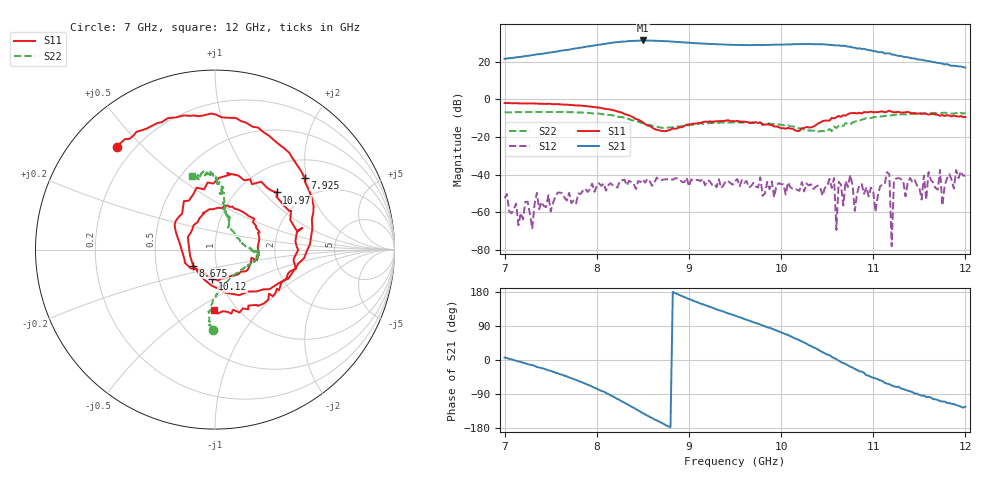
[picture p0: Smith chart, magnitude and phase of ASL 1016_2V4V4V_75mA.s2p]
!ASL 1016 Low Noise Amplifier S-parameter data 7-12 GHz
!Bias conditions Vd1=2V,Vd2=4V,Vd3=4V ; Ids = 75mA
!Agilent Technologies,N5230A,US43500341,A.06.01.05
!Agilent N5230A: A.06.01.05
!Date: Wednesday, October 04, 2006 13:12:58
!Correction: S11(Full 2 Port(1,2)) S21(Full 2 Port(1,2)) S12(Full 2 Port(1,2)) S22(Full 2 Port(1,2))
!S2P File: Measurements: S11, S21, S12, S22:
# Hz S  dB  R 50
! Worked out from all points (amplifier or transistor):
!   201 points, 7 GHz to 12 GHz, reference 50 ohm
!   highest |S21| = 31.2 dB at 8.5 GHz (marker M1)
!   |S21| within 3 dB of that: 7.931 GHz to 10.71 GHz (2.775 GHz wide, 29.8 % of centre)
!   unconditionally stable (mu >= 1): start of sweep to end of sweep
!   at 7.825 GHz: K = 3.33, MAG = 30.7 dB, |S12| = -50.2 dB
!   at 9.5 GHz: K = 2.53, MAG = 29.3 dB, |S12| = -43.5 dB
!   at 12 GHz: K = 5.47, MAG = 18.3 dB, |S12| = -40.5 dB
!   S11 on the Smith chart (normalised r, x): 7 GHz: 0.14, +0.42; 7.925 GHz: 1.43, +1.95; 8.675 GHz: 0.77, -0.14; 10.12 GHz: 0.92, -0.31; 10.97 GHz: 1.47, +1.20; 12 GHz: 0.79, -0.60
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7e9  -2.06 133.5  21.47 6.2  -52.53 164.1  -6.95 -91.5
7.425e9  -2.52 97.0  24.22 -22.6  -56.60 -127.1  -6.71 -91.3
7.85e9  -3.51 49.7  27.58 -59.5  -48.46 -156.3  -7.05 -92.2
7.925e9  -3.87 38.8  28.11 -67.4  -47.80 -179.0  -7.32 -93.1
8.075e9  -4.95 17.4  29.30 -83.5  -44.60 -153.8  -7.99 -94.6
8.2e9  -6.05 -5.5  30.20 -99.8  -46.45 156.1  -8.70 -94.6
8.35e9  -8.51 -36.0  30.85 -119.2  -43.22 160.0  -10.44 -92.8
8.5e9  -12.21 -77.2  31.17 -140.1  -42.46 155.5  -12.75 -83.8
8.675e9  -16.45 -143.5  30.99 -162.5  -42.69 140.4  -14.83 -63.3
8.825e9  -15.55 155.0  30.56 179.4  -42.74 138.3  -15.01 -42.4
9.05e9  -12.88 97.9  29.77 155.9  -43.07 115.0  -13.52 -22.4
9.5e9  -11.74 28.4  28.82 117.4  -43.48 111.7  -12.50 -7.9
9.825e9  -13.43 -19.1  28.82 88.8  -49.92 89.4  -13.13 -3.2
1.0125e10  -15.65 -95.1  29.14 60.3  -47.37 87.4  -14.31 3.6
1.035e10  -14.52 178.7  29.20 33.7  -47.64 56.9  -16.66 25.0
1.0625e10  -8.87 106.6  28.60 -1.6  -43.76 43.8  -14.11 65.1
1.075e10  -7.41 78.5  27.84 -17.9  -40.22 -71.1  -13.39 74.5
1.0975e10  -6.58 42.8  25.97 -44.8  -46.84 -93.9  -10.00 79.9
1.1175e10  -6.02 14.0  24.35 -64.1  -39.85 -75.8  -8.75 88.2
1.12e10  -6.62 12.0  23.75 -67.2  -77.93 -161.9  -8.48 86.4
1.1525e10  -7.78 -32.2  20.90 -94.0  -53.23 53.3  -7.53 91.4
1.2e10  -9.42 -91.1  16.80 -123.2  -40.51 -171.8  -7.30 107.3
